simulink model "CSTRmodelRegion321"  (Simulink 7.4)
settings: Solver=ode15s  StartTime=0.0  StopTime=Tend  RelTol=1e-6
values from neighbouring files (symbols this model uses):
  cain = 2    [runDynSim321.m]    (also in sf_CSTR.m = cInVec(1))
  cbin = 1.5    [runDynSim321.m]    (also in sf_CSTR.m = cInVec(2))
undefined symbols (not defined in the file or in its folder): sigbuilder_block, Tuninpars, u0
libraries: simulink_extras x5

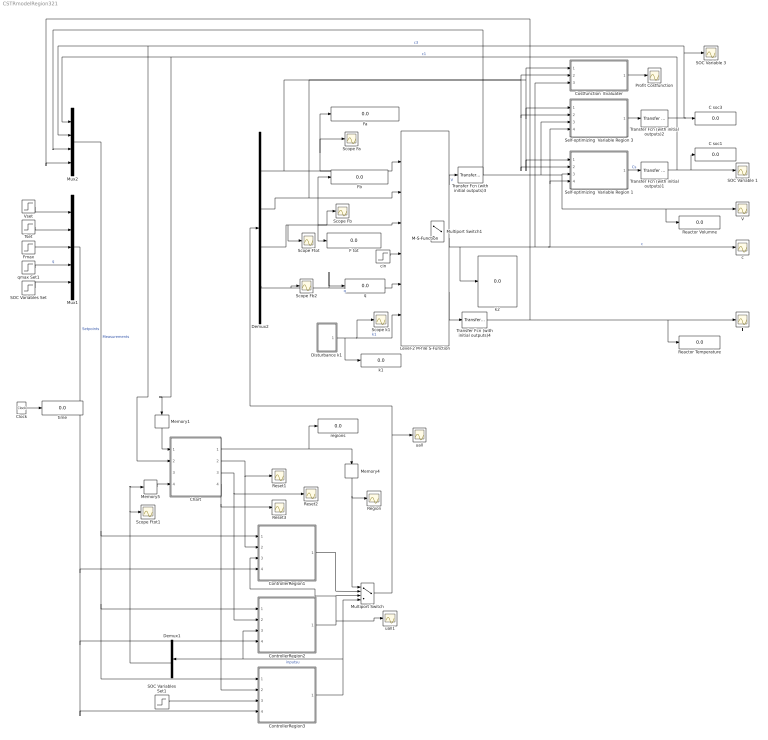
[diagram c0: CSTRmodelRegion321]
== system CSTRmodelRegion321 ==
  C soc1 : Display
  C soc3 : Display
  Chart : Stateflow chart
  Clock : Clock
  ControllerRegion1 : Subsystem
  ControllerRegion2 : Subsystem
  ControllerRegion3 : Subsystem
  Costfunction  Evaluater : Subsystem
  Demux1 : Demux
  Demux2 : Demux
  Disturbance k1 : Subsystem
  F tot : Display
  Fa : Display
  Fb : Display
  Fmax : Step  Time=0  Before=22  After=22  SampleTime=0
  Level-2 M-file S-Function : M-S-Function  FunctionName=sf_CSTR
  Memory1 : Memory  X0=3
  Memory4 : Memory  X0=3
  Memory5 : Memory  X0=3
  Multiport Switch : MultiPortSwitch  OutDataType=fixdt(1, 16)  OutScaling=2^0
  Multiport Switch1 : MultiPortSwitch  OutDataType=fixdt(1, 16)  OutScaling=2^0
  Mux1 : Mux  Inputs=5
  Mux2 : Mux
  Profit Costfunction : Scope
  Reactor Temperature : Display
  Reactor Volumne : Display
  Region : Scope
  Reset1 : Scope
  Reset2 : Scope
  Reset3 : Scope
  SOC Variable 1 : Scope
  SOC Variable 3 : Scope
  SOC Variables Set : Step  Time=0  After=0  SampleTime=0
  SOC Variables Set1 : Step  Time=0  Before=u0  After=u0  SampleTime=0
  Scope Fa : Scope
  Scope Fb : Scope
  Scope Fb2 : Scope
  Scope Ftot : Scope
  Scope Ftot1 : Scope
  Scope k1 : Scope
  Self-optimizing  Variable Region 1 : Stateflow chart
  Self-optimizing  Variable Region 3 : Stateflow chart
  T : Scope
  Transfer Fcn (with initial outputs)1 : simulink_extras/Additional Linear/Transfer Fcn (with initial outputs)  SystemSampleTime=-1  N=[1]  D="[1  1]"  Y0=11.24  U0=11.24
  Transfer Fcn (with initial outputs)2 : simulink_extras/Additional Linear/Transfer Fcn (with initial outputs)  SystemSampleTime=-1  N=[1]  D="[1  1]"  Y0=0  U0=0
  Transfer Fcn (with initial outputs)3 : simulink_extras/Additional Linear/Transfer Fcn (with initial outputs)  SystemSampleTime=-1  N=[1]  D="[1  1]"  Y0=500  U0=500
  Transfer Fcn (with initial outputs)4 : simulink_extras/Additional Linear/Transfer Fcn (with initial outputs)  SystemSampleTime=-1  N=[1]  D="[1  1]"  Y0=350  U0=350
  Tset : Step  Time=250  Before=350  After=350  SampleTime=0
  V : Scope
  Vset : Step  Time=0  Before=500  After=500  SampleTime=0
  c : Scope
  cin : Step  Time=0  Before=[cain cbin 0 0]  After=[cain cbin 0 0]  SampleTime=0
  k1 : Display
  k2 : Display
  q : Display
  qmax Set1 : Step  Time=0  Before=1000  After=1000  SampleTime=0
  regions : Display
  time : Display
  uall : Scope
  uall1 : Scope
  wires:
  cin/1 -> Level-2 M-file S-Function/4
  Level-2 M-file S-Function/1 -> Transfer Fcn (with initial outputs)3/1  "V"
  Level-2 M-file S-Function/2 -> Costfunction  Evaluater/3(Concentrations), c/1, Self-optimizing  Variable Region 1/4(cVector), Self-optimizing  Variable Region 3/4(cVector), k2/1  "c"
  Level-2 M-file S-Function/3 -> Transfer Fcn (with initial outputs)4/1  "T"
  Costfunction  Evaluater/1(Objective) -> Profit Costfunction/1
  Self-optimizing  Variable Region 1/1(cs) -> Transfer Fcn (with initial outputs)1/1  "Cs"
  Disturbance k1/1(Out1) -> Scope k1/1, Level-2 M-file S-Function/6, k1/1  "k1"
  qmax Set1/1 -> Mux1/4  "q"
  Vset/1 -> Mux1/1
  Fmax/1 -> Mux1/3
  Tset/1 -> Mux1/2
  Mux2/1 -> ControllerRegion3/1(In1), ControllerRegion2/1(In1), ControllerRegion1/1(In1)  "Measurements"
  Demux2/1 -> Costfunction  Evaluater/1(Fa), Self-optimizing  Variable Region 1/1(Fa), Self-optimizing  Variable Region 3/1(Fa), Level-2 M-file S-Function/1, Fa/1, Scope Fa/1
  Demux2/2 -> Costfunction  Evaluater/2(Fb), Self-optimizing  Variable Region 1/2(Fb), Self-optimizing  Variable Region 3/2(Fb), Scope Fb/1, Level-2 M-file S-Function/2, Fb/1
  Demux2/3 -> Level-2 M-file S-Function/3, F tot/1, Scope Ftot/1
  Demux2/4 -> Level-2 M-file S-Function/5, q/1, Scope Fb2/1  "q"
  Mux1/1 -> ControllerRegion3/4(In4), ControllerRegion2/4(In4), ControllerRegion1/4(In4)  "Setpoints"
  Transfer Fcn (with initial outputs)1/1 -> SOC Variable 1/1, C soc1/1, Mux2/1, Memory1/1  "c1"
  Chart/1(R) -> regions/1, Memory4/1
  Self-optimizing  Variable Region 3/1(cs) -> Transfer Fcn (with initial outputs)2/1
  SOC Variables Set/1 -> Mux1/5
  Transfer Fcn (with initial outputs)2/1 -> C soc3/1, SOC Variable 3/1, Mux2/2, Chart/2(c3)  "c3"
  ControllerRegion1/1(Out2) -> Multiport Switch/2
  ControllerRegion2/1(Out2) -> Multiport Switch/3, ControllerRegion1/3(In3), uall1/1
  ControllerRegion3/1(Out2) -> Multiport Switch/4, Demux1/1, ControllerRegion2/3(In3)  "inputsu"
  Multiport Switch/1 -> Demux2/1, uall/1
  SOC Variables Set1/1 -> ControllerRegion3/3(In3)
  Demux1/3 -> Scope Ftot1/1, Memory5/1
  Memory4/1 -> Multiport Switch/1, Region/1
  Memory5/1 -> Chart/4(Ftot)
  Memory1/1 -> Chart/1(c1)
  Chart/2(reset1) -> ControllerRegion1/2(In2), Reset1/1
  Chart/3(reset2) -> ControllerRegion2/2(In2), Reset2/1
  Chart/4(reset3) -> ControllerRegion3/2(In2), Reset3/1
  Clock/1 -> time/1
  Transfer Fcn (with initial outputs)3/1 -> Self-optimizing  Variable Region 1/3(V), V/1, Reactor Volumne/1, Self-optimizing  Variable Region 3/3(V), Mux2/3
  Transfer Fcn (with initial outputs)4/1 -> T/1, Reactor Temperature/1, Mux2/4

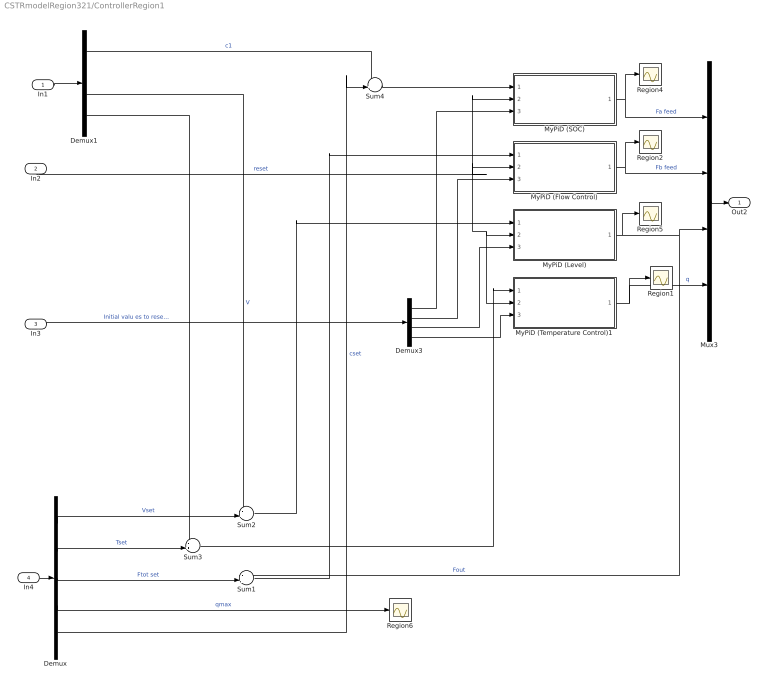
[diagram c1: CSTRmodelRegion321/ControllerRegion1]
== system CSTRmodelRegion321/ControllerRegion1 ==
  In1 : Inport
  In2 : Inport  Port=2
  In3 : Inport  Port=3
  In4 : Inport  Port=4
  Demux : Demux  Outputs=5
  Demux1 : Demux
  Demux3 : Demux
  Mux3 : Mux
  MyPiD (Flow Control) : Subsystem  mask{Kp=Tuninpars.Reg1.FlowController.Kp, TauiInv=Tuninpars.Reg1.FlowController.TauiInv, UB=1000, LB=1}
      mask prompts: Kp "Proportional Gain Kp"; TauiInv "Inverse Integral time"; UB "Upper bound"; LB "Lower bound"
  MyPiD (Level) : Subsystem  mask{Kp=Tuninpars.Reg1.LevelController.Kp, TauiInv=Tuninpars.Reg1.LevelController.TauiInv, UB=[40], LB=2}
      mask prompts: Kp "Proportional Gain Kp"; TauiInv "Inverse Integral time"; UB "Upper bound"; LB "Lower bound"
  MyPiD (SOC) : Subsystem  mask{Kp=Tuninpars.Reg1.SocController.Kp, TauiInv=Tuninpars.Reg1.SocController.TauiInv, UB=inf, LB=2}
      mask prompts: Kp "Proportional Gain Kp"; TauiInv "Inverse Integral time"; UB "Upper bound"; LB "Lower bound"
  MyPiD (Temperature Control)1 : Subsystem  mask{Kp=Tuninpars.Reg1.TempController.Kp, TauiInv=Tuninpars.Reg1.TempController.TauiInv, UB=1000, LB=1}
      mask prompts: Kp "Proportional Gain Kp"; TauiInv "Inverse Integral time"; UB "Upper bound"; LB "Lower bound"
  Region{1..2,4..6} (5 alike) : Scope
  Sum{1..4} (4 alike) : Sum  Inputs=-+|  OutDataType=fixdt(1, 16)  OutScaling=2^0
  Out2 : Outport
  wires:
  Sum4/1 -> MyPiD (SOC)/1(In1)
  MyPiD (Flow Control)/1(Out1) -> Region2/1, Mux3/2  "Fb feed"
  Sum2/1 -> MyPiD (Level)/1(In1)
  MyPiD (Level)/1(Out1) -> Region5/1, Mux3/3, Sum1/1  "Fout"
  Sum3/1 -> MyPiD (Temperature Control)1/1(In1)
  Demux1/1 -> Sum4/1  "c1"
  MyPiD (SOC)/1(Out1) -> Region4/1, Mux3/1  "Fa feed"
  Demux/2 -> Sum3/2  "Tset"
  Demux/1 -> Sum2/2  "Vset"
  Demux3/1 -> MyPiD (SOC)/3(In3)
  Demux3/2 -> MyPiD (Flow Control)/3(In3)
  In1/1 -> Demux1/1
  In2/1 -> MyPiD (Level)/2(In2), MyPiD (Temperature Control)1/2(In2), MyPiD (Flow Control)/2(In2), MyPiD (SOC)/2(In2)  "reset"
  In3/1 -> Demux3/1  "Initial valu es to reset to"
  In4/1 -> Demux/1
  Mux3/1 -> Out2/1
  Demux/4 -> Region6/1  "qmax"
  Demux/5 -> Sum4/2  "cset"
  Demux1/4 -> Sum3/1  "T"
  Demux1/3 -> Sum2/1  "V"
  Demux1/2 -> ?  "c3"
  Demux3/3 -> MyPiD (Level)/3(In3)
  MyPiD (Temperature Control)1/1(Out1) -> Mux3/4, Region1/1  "q"
  Demux3/4 -> MyPiD (Temperature Control)1/3(In3)
  Demux/3 -> Sum1/2  "Ftot set"
  Sum1/1 -> MyPiD (Flow Control)/1(In1)

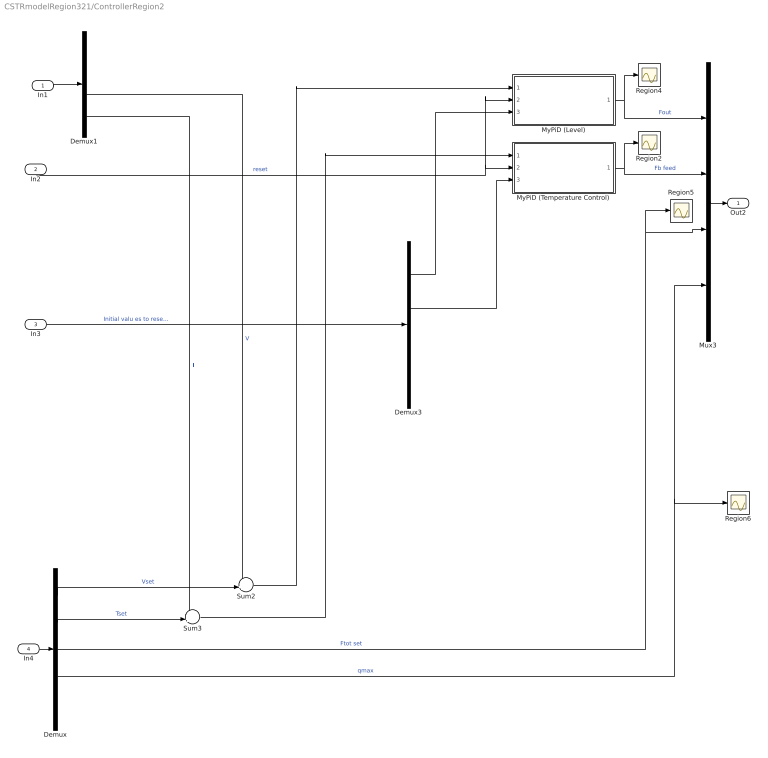
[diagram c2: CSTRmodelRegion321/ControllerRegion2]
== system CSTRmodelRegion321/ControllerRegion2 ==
  In1 : Inport
  In2 : Inport  Port=2
  In3 : Inport  Port=3
  In4 : Inport  Port=4
  Demux : Demux  Outputs=5
  Demux1 : Demux
  Demux3 : Demux
  Mux3 : Mux
  MyPiD (Level) : Subsystem  mask{Kp=Tuninpars.Reg2.LevelController.Kp, TauiInv=Tuninpars.Reg2.LevelController.TauiInv, UB=10, LB=4}
      mask prompts: Kp "Proportional Gain Kp"; TauiInv "Inverse Integral time"; UB "Upper bound"; LB "Lower bound"
  MyPiD (Temperature Control) : Subsystem  mask{Kp=Tuninpars.Reg2.TempController.Kp, TauiInv=Tuninpars.Reg2.TempController.TauiInv, UB=20, LB=5}
      mask prompts: Kp "Proportional Gain Kp"; TauiInv "Inverse Integral time"; UB "Upper bound"; LB "Lower bound"
  Region{2,4..6} (4 alike) : Scope
  Sum2 : Sum  Inputs=-+|  OutDataType=fixdt(1, 16)  OutScaling=2^0
  Sum3 : Sum  Inputs=-+|  OutDataType=fixdt(1, 16)  OutScaling=2^0
  Out2 : Outport
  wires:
  Demux3/3 -> ?
  Demux1/3 -> Sum2/1  "V"
  Demux1/4 -> Sum3/1  "T"
  Demux/3 -> Mux3/3, Region5/1  "Ftot set"
  Demux/4 -> Mux3/4, Region6/1  "qmax"
  Mux3/1 -> Out2/1
  In4/1 -> Demux/1
  In3/1 -> Demux3/1  "Initial valu es to reset to"
  In2/1 -> MyPiD (Level)/2(In2), MyPiD (Temperature Control)/2(In2)  "reset"
  In1/1 -> Demux1/1
  Demux3/2 -> MyPiD (Temperature Control)/3(In3)
  Demux3/1 -> MyPiD (Level)/3(In3)
  Demux/1 -> Sum2/2  "Vset"
  Demux/2 -> Sum3/2  "Tset"
  MyPiD (Level)/1(Out1) -> Region4/1, Mux3/1  "Fout"
  Demux1/1 -> ?  "c1"
  Sum3/1 -> MyPiD (Temperature Control)/1(In1)
  Sum2/1 -> MyPiD (Level)/1(In1)
  MyPiD (Temperature Control)/1(Out1) -> Region2/1, Mux3/2  "Fb feed"
  Demux1/2 -> ?  "c3"

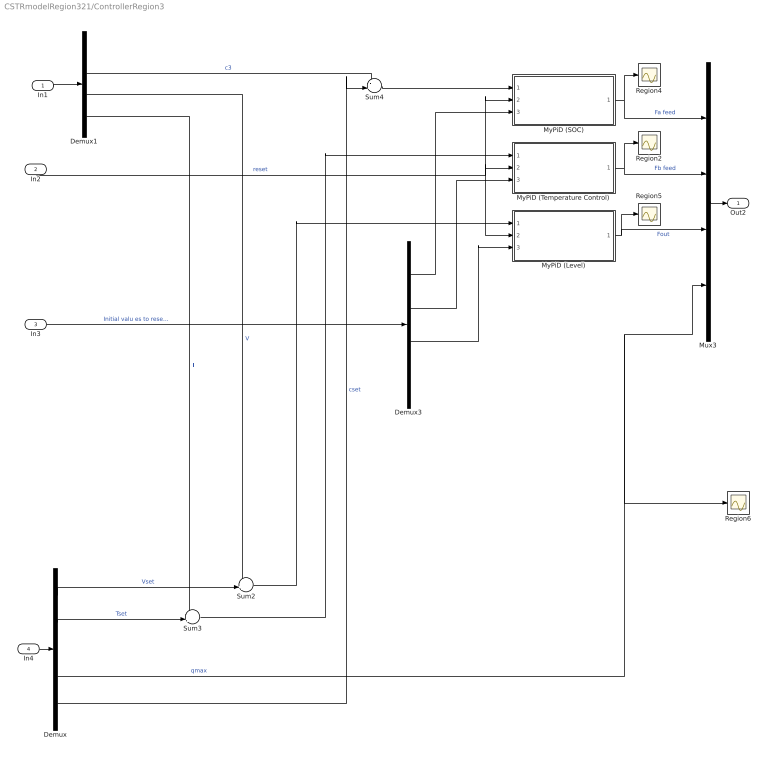
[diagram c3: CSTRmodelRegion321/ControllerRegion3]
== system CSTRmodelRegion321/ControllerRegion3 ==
  In1 : Inport
  In2 : Inport  Port=2
  In3 : Inport  Port=3
  In4 : Inport  Port=4
  Demux : Demux  Outputs=5
  Demux1 : Demux
  Demux3 : Demux
  Mux3 : Mux
  MyPiD (Level) : Subsystem  mask{Kp=Tuninpars.Reg3.LevelController.Kp, TauiInv=Tuninpars.Reg3.LevelController.TauiInv, UB=[40], LB=2}
      mask prompts: Kp "Proportional Gain Kp"; TauiInv "Inverse Integral time"; UB "Upper bound"; LB "Lower bound"
  MyPiD (SOC) : Subsystem  mask{Kp=Tuninpars.Reg3.SocController.Kp, TauiInv=Tuninpars.Reg3.SocController.TauiInv, UB=inf, LB=2}
      mask prompts: Kp "Proportional Gain Kp"; TauiInv "Inverse Integral time"; UB "Upper bound"; LB "Lower bound"
  MyPiD (Temperature Control) : Subsystem  mask{Kp=Tuninpars.Reg3.TempController.Kp, TauiInv=Tuninpars.Reg3.TempController.TauiInv, UB=1000, LB=1}
      mask prompts: Kp "Proportional Gain Kp"; TauiInv "Inverse Integral time"; UB "Upper bound"; LB "Lower bound"
  Region{2,4..6} (4 alike) : Scope
  Sum2 : Sum  Inputs=-+|  OutDataType=fixdt(1, 16)  OutScaling=2^0
  Sum3 : Sum  Inputs=-+|  OutDataType=fixdt(1, 16)  OutScaling=2^0
  Sum4 : Sum  Inputs=-+|  OutDataType=fixdt(1, 16)  OutScaling=2^0
  Out2 : Outport
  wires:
  Sum4/1 -> MyPiD (SOC)/1(In1)
  MyPiD (Temperature Control)/1(Out1) -> Mux3/2, Region2/1  "Fb feed"
  Sum2/1 -> MyPiD (Level)/1(In1)
  MyPiD (Level)/1(Out1) -> Region5/1, Mux3/3  "Fout"
  Sum3/1 -> MyPiD (Temperature Control)/1(In1)
  Demux1/1 -> ?  "c1"
  MyPiD (SOC)/1(Out1) -> Mux3/1, Region4/1  "Fa feed"
  Demux/2 -> Sum3/2  "Tset"
  Demux/1 -> Sum2/2  "Vset"
  Demux3/1 -> MyPiD (SOC)/3(In3)
  Demux3/2 -> MyPiD (Temperature Control)/3(In3)
  In1/1 -> Demux1/1
  In2/1 -> MyPiD (Temperature Control)/2(In2), MyPiD (Level)/2(In2), MyPiD (SOC)/2(In2)  "reset"
  In3/1 -> Demux3/1  "Initial valu es to reset to"
  In4/1 -> Demux/1
  Mux3/1 -> Out2/1
  Demux/4 -> Region6/1, Mux3/4  "qmax"
  Demux/5 -> Sum4/2  "cset"
  Demux/3 -> ?  "Ftot set"
  Demux1/4 -> Sum3/1  "T"
  Demux1/3 -> Sum2/1  "V"
  Demux1/2 -> Sum4/1  "c3"
  Demux3/3 -> MyPiD (Level)/3(In3)

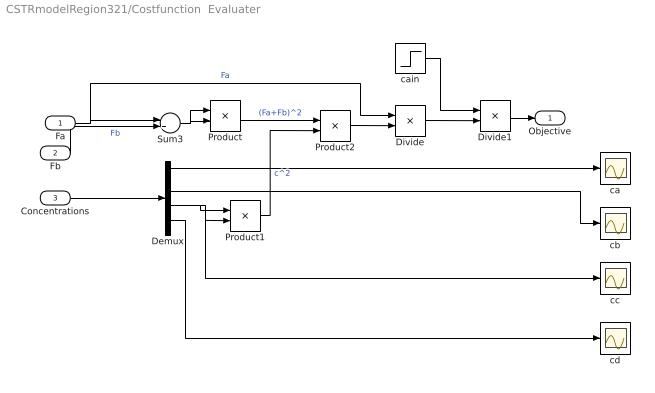
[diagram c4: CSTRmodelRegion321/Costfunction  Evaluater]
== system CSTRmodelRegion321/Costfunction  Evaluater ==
  Fa : Inport
  Fb : Inport  Port=2
  Concentrations : Inport  Port=3
  Demux : Demux
  Divide : Product  Inputs=/*  OutDataType=fixdt(1, 16)  OutScaling=2^-10
  Divide1 : Product  Inputs=/*  OutDataType=fixdt(1, 16)  OutScaling=2^-10
  Product : Product  OutDataType=fixdt(1, 16)  OutScaling=2^0
  Product1 : Product  OutDataType=fixdt(1, 16)  OutScaling=2^0
  Product2 : Product  OutDataType=fixdt(1, 16)  OutScaling=2^0
  Sum3 : Sum  Inputs=|++  OutDataType=fixdt(1, 16)  OutScaling=2^0
  ca : Scope
  cain : Step  Before=cain  After=cain  SampleTime=0
  cb : Scope
  cc : Scope
  cd : Scope
  Objective : Outport
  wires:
  Sum3/1 -> Product/1, Product/2
  Demux/3 -> Product1/1, Product1/2, cc/1
  Product/1 -> Product2/1  "(Fa+Fb)^2"
  Product1/1 -> Product2/2  "c^2"
  Product2/1 -> Divide/2
  Divide/1 -> Divide1/2
  cain/1 -> Divide1/1
  Fa/1 -> Sum3/1, Divide/1  "Fa"
  Fb/1 -> Sum3/2  "Fb"
  Concentrations/1 -> Demux/1
  Divide1/1 -> Objective/1
  Demux/1 -> ca/1
  Demux/2 -> cb/1
  Demux/4 -> cd/1

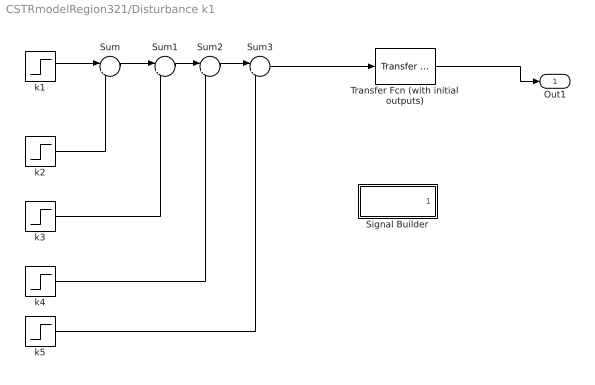
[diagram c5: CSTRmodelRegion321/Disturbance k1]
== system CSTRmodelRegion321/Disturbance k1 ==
  Signal Builder : Subsystem  Tag=STV Subsys  LoadFcn=sigbuilder_block('load');  StartFcn=sigbuilder_block('start');  StopFcn=sigbuilder_block('stop');  ClipboardFcn=sigbuilder_block('clipboard');
  Sum{,1..3} (4 alike) : Sum  Inputs=|+-  OutDataType=fixdt(1, 16)  OutScaling=2^0
  Transfer Fcn (with initial outputs) : simulink_extras/Additional Linear/Transfer Fcn (with initial outputs)  SystemSampleTime=-1  N=[1]  D="[25  1]"  Y0=1.5  U0=0
  k1 : Step  Time=200  Before=1.5  After=1.1  SampleTime=0
  k2 : Step  Time=400  After=0.3  SampleTime=0
  k3 : Step  Time=600  After=0.1  SampleTime=0
  k4 : Step  Time=800  After=0.3  SampleTime=0
  k5 : Step  Time=1000  After=0.1  SampleTime=0
  Out1 : Outport
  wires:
  Transfer Fcn (with initial outputs)/1 -> Out1/1
  k1/1 -> Sum/1
  Sum/1 -> Sum1/1
  k2/1 -> Sum/2
  Sum1/1 -> Sum2/1
  k3/1 -> Sum1/2
  Sum2/1 -> Sum3/1
  k4/1 -> Sum2/2
  Sum3/1 -> Transfer Fcn (with initial outputs)/1
  k5/1 -> Sum3/2

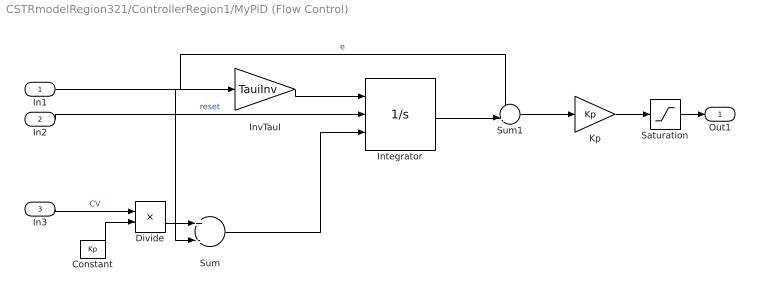
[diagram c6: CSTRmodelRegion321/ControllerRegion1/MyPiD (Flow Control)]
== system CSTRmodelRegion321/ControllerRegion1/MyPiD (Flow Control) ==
  In1 : Inport
  In2 : Inport  Port=2
  In3 : Inport  Port=3
  Constant : Constant  Value=Kp  OutDataType=fixdt(1, 16)  OutScaling=2^0
  Divide : Product  Inputs=*/  OutDataType=fixdt(1, 16)  OutScaling=2^-10
  Integrator : Integrator  ExternalReset=rising  InitialConditionSource=external
  InvTauI : Gain  Gain=TauiInv  ParameterDataType=fixdt(1, 16)  ParameterScaling=2^0  OutDataType=fixdt(1, 16)  OutScaling=2^0
  Kp : Gain  Gain=Kp  ParameterDataType=fixdt(1, 16)  ParameterScaling=2^0  OutDataType=fixdt(1, 16)  OutScaling=2^0
  Saturation : Saturate  UpperLimit=UB  LowerLimit=LB  LinearizeAsGain=off  OutDataType=SaturationOutDataTypeStr
  Sum : Sum  Inputs=+-  OutDataType=fixdt(1, 16)  OutScaling=2^0
  Sum1 : Sum  Inputs=++|  OutDataType=fixdt(1, 16)  OutScaling=2^0
  Out1 : Outport
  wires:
  InvTauI/1 -> Integrator/1
  Sum1/1 -> Kp/1
  Integrator/1 -> Sum1/2
  Kp/1 -> Saturation/1
  In2/1 -> Integrator/2  "reset"
  In1/1 -> InvTauI/1, Sum1/1, Sum/2  "e"
  Saturation/1 -> Out1/1
  In3/1 -> Divide/1  "CV"
  Constant/1 -> Divide/2
  Divide/1 -> Sum/1
  Sum/1 -> Integrator/3

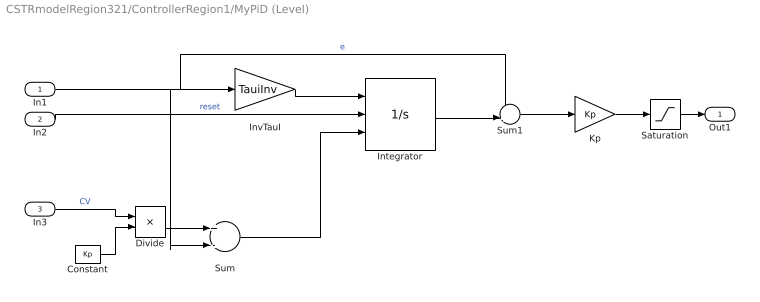
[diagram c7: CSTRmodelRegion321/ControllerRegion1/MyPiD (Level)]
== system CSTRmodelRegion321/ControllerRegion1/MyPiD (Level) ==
  In1 : Inport
  In2 : Inport  Port=2
  In3 : Inport  Port=3
  Constant : Constant  Value=Kp  OutDataType=fixdt(1, 16)  OutScaling=2^0
  Divide : Product  Inputs=*/  OutDataType=fixdt(1, 16)  OutScaling=2^-10
  Integrator : Integrator  ExternalReset=rising  InitialConditionSource=external
  InvTauI : Gain  Gain=TauiInv  ParameterDataType=fixdt(1, 16)  ParameterScaling=2^0  OutDataType=fixdt(1, 16)  OutScaling=2^0
  Kp : Gain  Gain=Kp  ParameterDataType=fixdt(1, 16)  ParameterScaling=2^0  OutDataType=fixdt(1, 16)  OutScaling=2^0
  Saturation : Saturate  UpperLimit=UB  LowerLimit=LB  LinearizeAsGain=off  OutDataType=SaturationOutDataTypeStr
  Sum : Sum  Inputs=+-  OutDataType=fixdt(1, 16)  OutScaling=2^0
  Sum1 : Sum  Inputs=++|  OutDataType=fixdt(1, 16)  OutScaling=2^0
  Out1 : Outport
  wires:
  InvTauI/1 -> Integrator/1
  Sum1/1 -> Kp/1
  Integrator/1 -> Sum1/2
  Kp/1 -> Saturation/1
  In2/1 -> Integrator/2  "reset"
  In1/1 -> InvTauI/1, Sum1/1, Sum/2  "e"
  Saturation/1 -> Out1/1
  In3/1 -> Divide/1  "CV"
  Constant/1 -> Divide/2
  Divide/1 -> Sum/1
  Sum/1 -> Integrator/3

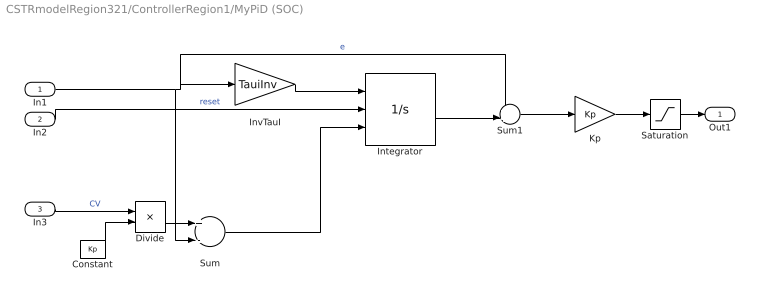
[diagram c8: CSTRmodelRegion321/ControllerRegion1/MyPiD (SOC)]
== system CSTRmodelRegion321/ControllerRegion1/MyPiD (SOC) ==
  In1 : Inport
  In2 : Inport  Port=2
  In3 : Inport  Port=3
  Constant : Constant  Value=Kp  OutDataType=fixdt(1, 16)  OutScaling=2^0
  Divide : Product  Inputs=*/  OutDataType=fixdt(1, 16)  OutScaling=2^-10
  Integrator : Integrator  ExternalReset=rising  InitialConditionSource=external
  InvTauI : Gain  Gain=TauiInv  ParameterDataType=fixdt(1, 16)  ParameterScaling=2^0  OutDataType=fixdt(1, 16)  OutScaling=2^0
  Kp : Gain  Gain=Kp  ParameterDataType=fixdt(1, 16)  ParameterScaling=2^0  OutDataType=fixdt(1, 16)  OutScaling=2^0
  Saturation : Saturate  UpperLimit=UB  LowerLimit=LB  LinearizeAsGain=off  OutDataType=SaturationOutDataTypeStr
  Sum : Sum  Inputs=+-  OutDataType=fixdt(1, 16)  OutScaling=2^0
  Sum1 : Sum  Inputs=++|  OutDataType=fixdt(1, 16)  OutScaling=2^0
  Out1 : Outport
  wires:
  InvTauI/1 -> Integrator/1
  Sum1/1 -> Kp/1
  Integrator/1 -> Sum1/2
  Kp/1 -> Saturation/1
  In2/1 -> Integrator/2  "reset"
  In1/1 -> InvTauI/1, Sum1/1, Sum/2  "e"
  Saturation/1 -> Out1/1
  In3/1 -> Divide/1  "CV"
  Constant/1 -> Divide/2
  Divide/1 -> Sum/1
  Sum/1 -> Integrator/3

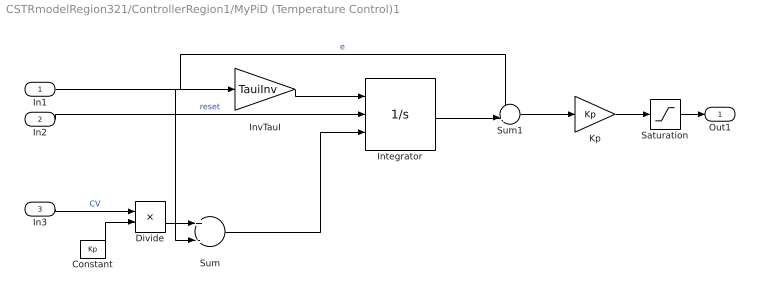
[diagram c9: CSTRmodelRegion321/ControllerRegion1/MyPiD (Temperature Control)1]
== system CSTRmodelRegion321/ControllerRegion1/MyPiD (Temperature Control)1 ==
  In1 : Inport
  In2 : Inport  Port=2
  In3 : Inport  Port=3
  Constant : Constant  Value=Kp  OutDataType=fixdt(1, 16)  OutScaling=2^0
  Divide : Product  Inputs=*/  OutDataType=fixdt(1, 16)  OutScaling=2^-10
  Integrator : Integrator  ExternalReset=rising  InitialConditionSource=external
  InvTauI : Gain  Gain=TauiInv  ParameterDataType=fixdt(1, 16)  ParameterScaling=2^0  OutDataType=fixdt(1, 16)  OutScaling=2^0
  Kp : Gain  Gain=Kp  ParameterDataType=fixdt(1, 16)  ParameterScaling=2^0  OutDataType=fixdt(1, 16)  OutScaling=2^0
  Saturation : Saturate  UpperLimit=UB  LowerLimit=LB  LinearizeAsGain=off  OutDataType=SaturationOutDataTypeStr
  Sum : Sum  Inputs=+-  OutDataType=fixdt(1, 16)  OutScaling=2^0
  Sum1 : Sum  Inputs=++|  OutDataType=fixdt(1, 16)  OutScaling=2^0
  Out1 : Outport
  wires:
  Sum/1 -> Integrator/3
  Divide/1 -> Sum/1
  Constant/1 -> Divide/2
  In3/1 -> Divide/1  "CV"
  Saturation/1 -> Out1/1
  In1/1 -> Sum/2, Sum1/1, InvTauI/1  "e"
  In2/1 -> Integrator/2  "reset"
  Kp/1 -> Saturation/1
  Integrator/1 -> Sum1/2
  Sum1/1 -> Kp/1
  InvTauI/1 -> Integrator/1

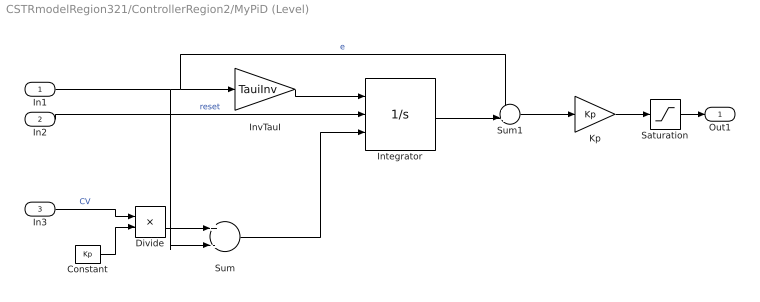
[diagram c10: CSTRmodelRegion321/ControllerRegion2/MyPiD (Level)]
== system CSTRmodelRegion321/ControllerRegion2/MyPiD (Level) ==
  In1 : Inport
  In2 : Inport  Port=2
  In3 : Inport  Port=3
  Constant : Constant  Value=Kp  OutDataType=fixdt(1, 16)  OutScaling=2^0
  Divide : Product  Inputs=*/  OutDataType=fixdt(1, 16)  OutScaling=2^-10
  Integrator : Integrator  ExternalReset=rising  InitialConditionSource=external
  InvTauI : Gain  Gain=TauiInv  ParameterDataType=fixdt(1, 16)  ParameterScaling=2^0  OutDataType=fixdt(1, 16)  OutScaling=2^0
  Kp : Gain  Gain=Kp  ParameterDataType=fixdt(1, 16)  ParameterScaling=2^0  OutDataType=fixdt(1, 16)  OutScaling=2^0
  Saturation : Saturate  UpperLimit=UB  LowerLimit=LB  LinearizeAsGain=off  OutDataType=SaturationOutDataTypeStr
  Sum : Sum  Inputs=+-  OutDataType=fixdt(1, 16)  OutScaling=2^0
  Sum1 : Sum  Inputs=++|  OutDataType=fixdt(1, 16)  OutScaling=2^0
  Out1 : Outport
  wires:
  Sum/1 -> Integrator/3
  Divide/1 -> Sum/1
  Constant/1 -> Divide/2
  In3/1 -> Divide/1  "CV"
  Saturation/1 -> Out1/1
  In1/1 -> Sum/2, Sum1/1, InvTauI/1  "e"
  In2/1 -> Integrator/2  "reset"
  Kp/1 -> Saturation/1
  Integrator/1 -> Sum1/2
  Sum1/1 -> Kp/1
  InvTauI/1 -> Integrator/1

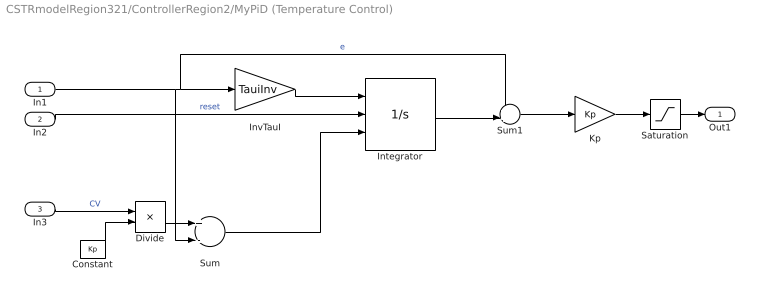
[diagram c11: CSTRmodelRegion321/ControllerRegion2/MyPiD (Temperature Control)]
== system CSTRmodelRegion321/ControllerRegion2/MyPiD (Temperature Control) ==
  In1 : Inport
  In2 : Inport  Port=2
  In3 : Inport  Port=3
  Constant : Constant  Value=Kp  OutDataType=fixdt(1, 16)  OutScaling=2^0
  Divide : Product  Inputs=*/  OutDataType=fixdt(1, 16)  OutScaling=2^-10
  Integrator : Integrator  ExternalReset=rising  InitialConditionSource=external
  InvTauI : Gain  Gain=TauiInv  ParameterDataType=fixdt(1, 16)  ParameterScaling=2^0  OutDataType=fixdt(1, 16)  OutScaling=2^0
  Kp : Gain  Gain=Kp  ParameterDataType=fixdt(1, 16)  ParameterScaling=2^0  OutDataType=fixdt(1, 16)  OutScaling=2^0
  Saturation : Saturate  UpperLimit=UB  LowerLimit=LB  LinearizeAsGain=off  OutDataType=SaturationOutDataTypeStr
  Sum : Sum  Inputs=+-  OutDataType=fixdt(1, 16)  OutScaling=2^0
  Sum1 : Sum  Inputs=++|  OutDataType=fixdt(1, 16)  OutScaling=2^0
  Out1 : Outport
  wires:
  Sum/1 -> Integrator/3
  Divide/1 -> Sum/1
  Constant/1 -> Divide/2
  In3/1 -> Divide/1  "CV"
  Saturation/1 -> Out1/1
  In1/1 -> Sum/2, Sum1/1, InvTauI/1  "e"
  In2/1 -> Integrator/2  "reset"
  Kp/1 -> Saturation/1
  Integrator/1 -> Sum1/2
  Sum1/1 -> Kp/1
  InvTauI/1 -> Integrator/1

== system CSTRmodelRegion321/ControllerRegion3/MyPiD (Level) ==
  In1 : Inport
  In2 : Inport  Port=2
  In3 : Inport  Port=3
  Constant : Constant  Value=Kp  OutDataType=fixdt(1, 16)  OutScaling=2^0
  Divide : Product  Inputs=*/  OutDataType=fixdt(1, 16)  OutScaling=2^-10
  Integrator : Integrator  ExternalReset=rising  InitialConditionSource=external
  InvTauI : Gain  Gain=TauiInv  ParameterDataType=fixdt(1, 16)  ParameterScaling=2^0  OutDataType=fixdt(1, 16)  OutScaling=2^0
  Kp : Gain  Gain=Kp  ParameterDataType=fixdt(1, 16)  ParameterScaling=2^0  OutDataType=fixdt(1, 16)  OutScaling=2^0
  Saturation : Saturate  UpperLimit=UB  LowerLimit=LB  LinearizeAsGain=off  OutDataType=SaturationOutDataTypeStr
  Sum : Sum  Inputs=+-  OutDataType=fixdt(1, 16)  OutScaling=2^0
  Sum1 : Sum  Inputs=++|  OutDataType=fixdt(1, 16)  OutScaling=2^0
  Out1 : Outport
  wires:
  InvTauI/1 -> Integrator/1
  Sum1/1 -> Kp/1
  Integrator/1 -> Sum1/2
  Kp/1 -> Saturation/1
  In2/1 -> Integrator/2  "reset"
  In1/1 -> InvTauI/1, Sum1/1, Sum/2  "e"
  Saturation/1 -> Out1/1
  In3/1 -> Divide/1  "CV"
  Constant/1 -> Divide/2
  Divide/1 -> Sum/1
  Sum/1 -> Integrator/3

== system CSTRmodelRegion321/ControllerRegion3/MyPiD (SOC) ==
  In1 : Inport
  In2 : Inport  Port=2
  In3 : Inport  Port=3
  Constant : Constant  Value=Kp  OutDataType=fixdt(1, 16)  OutScaling=2^0
  Divide : Product  Inputs=*/  OutDataType=fixdt(1, 16)  OutScaling=2^-10
  Integrator : Integrator  ExternalReset=rising  InitialConditionSource=external
  InvTauI : Gain  Gain=TauiInv  ParameterDataType=fixdt(1, 16)  ParameterScaling=2^0  OutDataType=fixdt(1, 16)  OutScaling=2^0
  Kp : Gain  Gain=Kp  ParameterDataType=fixdt(1, 16)  ParameterScaling=2^0  OutDataType=fixdt(1, 16)  OutScaling=2^0
  Saturation : Saturate  UpperLimit=UB  LowerLimit=LB  LinearizeAsGain=off  OutDataType=SaturationOutDataTypeStr
  Sum : Sum  Inputs=+-  OutDataType=fixdt(1, 16)  OutScaling=2^0
  Sum1 : Sum  Inputs=++|  OutDataType=fixdt(1, 16)  OutScaling=2^0
  Out1 : Outport
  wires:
  InvTauI/1 -> Integrator/1
  Sum1/1 -> Kp/1
  Integrator/1 -> Sum1/2
  Kp/1 -> Saturation/1
  In2/1 -> Integrator/2  "reset"
  In1/1 -> InvTauI/1, Sum1/1, Sum/2  "e"
  Saturation/1 -> Out1/1
  In3/1 -> Divide/1  "CV"
  Constant/1 -> Divide/2
  Divide/1 -> Sum/1
  Sum/1 -> Integrator/3

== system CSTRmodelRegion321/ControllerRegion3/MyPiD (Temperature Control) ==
  In1 : Inport
  In2 : Inport  Port=2
  In3 : Inport  Port=3
  Constant : Constant  Value=Kp  OutDataType=fixdt(1, 16)  OutScaling=2^0
  Divide : Product  Inputs=*/  OutDataType=fixdt(1, 16)  OutScaling=2^-10
  Integrator : Integrator  ExternalReset=rising  InitialConditionSource=external
  InvTauI : Gain  Gain=TauiInv  ParameterDataType=fixdt(1, 16)  ParameterScaling=2^0  OutDataType=fixdt(1, 16)  OutScaling=2^0
  Kp : Gain  Gain=Kp  ParameterDataType=fixdt(1, 16)  ParameterScaling=2^0  OutDataType=fixdt(1, 16)  OutScaling=2^0
  Saturation : Saturate  UpperLimit=UB  LowerLimit=LB  LinearizeAsGain=off  OutDataType=SaturationOutDataTypeStr
  Sum : Sum  Inputs=+-  OutDataType=fixdt(1, 16)  OutScaling=2^0
  Sum1 : Sum  Inputs=++|  OutDataType=fixdt(1, 16)  OutScaling=2^0
  Out1 : Outport
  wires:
  InvTauI/1 -> Integrator/1
  Sum1/1 -> Kp/1
  Integrator/1 -> Sum1/2
  Kp/1 -> Saturation/1
  In2/1 -> Integrator/2  "reset"
  In1/1 -> InvTauI/1, Sum1/1, Sum/2  "e"
  Saturation/1 -> Out1/1
  In3/1 -> Divide/1  "CV"
  Constant/1 -> Divide/2
  Divide/1 -> Sum/1
  Sum/1 -> Integrator/3

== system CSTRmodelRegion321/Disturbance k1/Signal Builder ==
  Demux : Demux  Tag=STV Demux  Outputs=1
  FromWs : FromWorkspace  Tag=STV FromWs  VariableName=tuvar  SampleTime=0  SigBuilderData=DataTag0  VnvData=DataTag1
  Signal 1 : Outport  Tag=STV Outport  OutDataType=fixdt(1, 16)  OutScaling=2^0
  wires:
  Demux/1 -> Signal 1/1
  FromWs/1 -> Demux/1

== matlab function Self-optimizing 
Variable Region 1 ==
function cs = SOCVariable1(Fa,Fb,V,cVector)


cain        =  2;
cbin        = 1.5;
Fmax        = 22;
k2          =  0.0140;
cb          =  cVector(2);

cs = (-cbin^2*Fa^2-Fa^2*cain*cbin+6*Fa*cain*k2*cb^2*V+2*Fa*cain*Fmax*cb-Fa*cain*Fmax*cbin+4*V*k2*cb^3*Fmax+4*V^2*k2^2*cb^4-2*cbin*Fmax^2*cb+Fmax^2*cb^2-4*V*k2*cb^2*cbin*Fmax+cbin^2*Fmax^2);
cs =cs/10;

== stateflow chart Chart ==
  state Region2/
    entry: 	R = 2;
    entry:	reset2 =0;
    during: 	R=2;
    during: 	reset2=1;
    exit:	reset2 =0;
  state Region1/
    entry: 	R =1;
    entry: 	reset1 =0;
    during: 	R=1;
    during: 	reset1 =1;
    exit:	reset1 =0;
  state Region3/
    entry: 	R = 3;
    entry:	reset3 =0;
    during: 	R=3;
    during: 	reset3=1;
    exit:	reset3 = 0;
  Region2 -> Region1 : [c1<=0.0001]
  (default) -> Region3
  Region3 -> Region2 : [Ftot>=22&t>20]

== matlab function Self-optimizing 
Variable Region 3 ==
function cs = SOCVariable3(Fa,Fb,V,cVector)


cain        =  2;
cbin        = 1.5;
Fmax        = 22;
k2          =  0.0140;
cb          =  cVector(2);
H1          = -70;
H2          = -50;
qmax        = 1e3;



ScaleFactor = 2.5;

cs = (-4*V*cb^2*k2*H2*Fa*cain*cbin*qmax*H1+Fa*cbin^2*qmax^2*H1+4*V^2*cb^4*k2^2*H2*Fa*cain*cbin*H1^2-4*V^2*cb^4*k2^2*H2^2*Fa*cain*cbin*H1-2*V*cb^2*k2*Fa*cain*cbin*H1^2*qmax-4*V*cb^2*k2*H2*Fa*cbin^2*H1*qmax-2*V*cb^2*k2*H2*Fa^2*cain*cbin^2*H1^2+8*V*cb^3*k2*H2*H1*Fa*cain*qmax-8*V^2*cb^4*k2^2*H2*cbin*H1*qmax-12*V^2*cb^4*k2^2*Fa*H2^2*cbin^2*H1-8*V^2*cb^5*k2^2*H2*Fa*cain*H1^2+8*V^2*cb^5*k2^2*H2^2*H1*Fa*cain+8*V^2*cb^5*k2^2*Fa*H2^2*cbin*H1-qmax^3*cbin+2*cb*qmax^3-H1*cbin*Fa*cain*qmax^2+2*cb*Fa*cain*qmax^2*H1+Fa^2*cain*cbin^2*H1^2*qmax-2*cb*Fa*cbin*qmax^2*H1+8*V*cb^3*k2*H2*qmax^2+8*V^2*cb^5*k2^2*H2^2*qmax+8*V^3*cb^6*k2^3*H2^3*cbin-2*cb*Fa^2*cain*cbin*H1^2*qmax-2*V*cb^2*k2*H1*qmax^2*cbin-2*V*cb^2*k2*H2*qmax^2*cbin+4*V^2*cb^4*k2^2*H2^2*cbin*qmax-8*V^3*cb^6*k2^3*H2^2*cbin*H1)/(H1^2*H2*Fa*Fb);
%cs=cs/ScaleFactor;
